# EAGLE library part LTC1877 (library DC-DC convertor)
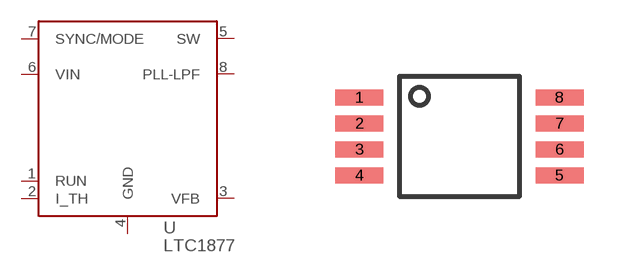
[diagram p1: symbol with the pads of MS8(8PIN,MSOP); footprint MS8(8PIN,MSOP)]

Designator prefix U

## LTC1877MSOP  [MS8(8PIN,MSOP)]
1  RUN
2  I_TH
3  VFB
4  GND
5  SW
6  VIN
7  SYNC/MODE
8  PLL-LPF

## Footprint MS8(8PIN,MSOP) (pad centres in mm)
MS8 package ; MSOP 8Pin ( 0.65mm pitch)
smd 1.2 x 0.4: 1 -2.5,0.975; 2 -2.5,0.325; 3 -2.5,-0.325; 4 -2.5,-0.975; 5 2.5,-0.975; 6 2.5,-0.325; 7 2.5,0.325; 8 2.5,0.975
